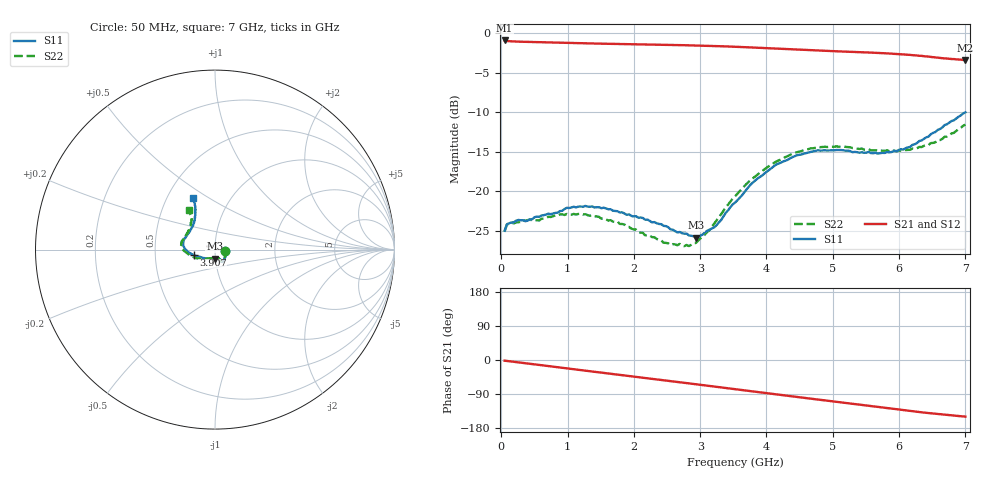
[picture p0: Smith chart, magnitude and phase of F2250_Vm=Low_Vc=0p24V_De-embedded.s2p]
! Integrated Device Technology
! Corporate Headquarters
! 6024 Silver Creek Valley Road
! San Jose, CA 95138  USA
! Phone:  1-408-284-8200
! Toll Free:  1-800-223-1366
! Webpage:  http://www.idt.com/
! Timing and RF Division
! 515 Groton Road, Suite 102
! Westford, MA 01886-6024
! Device:  F2250
! Description: Voltage Variable RF Attenuator
! Frequency:  50.0 -  6000.00 MHz
! Package:  3x3 mm Thin QFN Plastic Package: 16 pin
! Ports:  2 RF, 3 DC
!  Pin  1  = GND
!  Pin  2  = NC
!  Pin  3  = RF1  = Port 1
!  Pin  4  = NC
!  Pin  5  = GND
!  Pin  6  = GND
!  Pin  7  = GND
!  Pin  8  = GND
!  Pin  9  = NC
!  Pin 10  = RF2  = Port 2
!  Pin 11  = NC
!  Pin 12  = GND
!  Pin 13  = GND
!  Pin 14  = VCNTRL
!  Pin 15  = VDD
!  Pin 16  = VMODE
! Vcntrl:  0.240 Volts
! Vmode:  +0.000 Volts
! Vdd:  +3.30  Volts
! Current:  1.109 mA
! Data:  The device was measured on a the F2250 evaluation board which has
!  individual transmission lines to the RF pins.  Data was collected
!  using a calibrated network analyzer.  The evaluation board was
!  de-embedded using a TRL calibration technique.
!  The reference plane is the edge of the package pin.
! Misc:  SN 10
!  Action Tracker AT0258
! Date Measured:  2014-11-26
! Date:  2015-10-15  MJV
! Note:
!  Integrated Device Technology supplies this data as a sample of measured
!  data at the package pin for this product.  Your particular data for this
!  product may vary.
!  Data was taken at 25 degrees C.
!  Integrated Device Technology reserves the right to change this data at anytime.
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# GHz S dB R 50
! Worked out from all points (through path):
!   201 points, 50 MHz to 7 GHz, reference 50 ohm
!   highest |S21| = -0.93 dB at 50 MHz (marker M1); lowest = -3.4 dB at 7 GHz (marker M2)
!   group delay of S21, straight-line fit = 60 ps
!   lowest |S11| = -25.9 dB at 2.934 GHz (marker M3), VSWR 1.11, Z = 49.6 - j5.04 ohm
!   |S11| at or under -10 dB: start of sweep to end of sweep
!   |S22| runs from -27.0 to -11.6 dB; largest |S21 - S12| = 0.00036
!   S11 on the Smith chart (normalised r, x): 50 MHz: 1.12, -0.02; 3.907 GHz: 0.79, -0.05; 7 GHz: 0.67, +0.43
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0.05  -25.02 -9.6  -0.93 -1.8  -0.93 -1.8  -25.14 -10.1
0.08475  -24.20 -9.5  -1.00 -2.5  -1.00 -2.5  -24.26 -9.3
0.15425  -23.97 -11.8  -1.05 -4.0  -1.04 -4.0  -24.02 -11.0
0.57125  -23.26 -29.9  -1.15 -13.1  -1.15 -13.1  -23.74 -30.3
0.884  -22.55 -45.6  -1.21 -19.9  -1.21 -19.9  -22.98 -46.7
1.2315  -21.99 -55.8  -1.29 -27.4  -1.29 -27.4  -22.98 -59.6
1.75275  -22.56 -62.5  -1.38 -38.4  -1.38 -38.4  -23.86 -66.6
2.37825  -24.17 -63.3  -1.47 -51.8  -1.47 -51.8  -26.19 -67.9
2.552  -24.85 -67.5  -1.50 -55.6  -1.49 -55.6  -26.84 -73.4
2.83  -25.63 -82.8  -1.55 -61.7  -1.55 -61.7  -26.97 -92.7
2.93425  -25.89 -91.9  -1.57 -64.0  -1.57 -64.0  -26.58 -101.5
3.21225  -24.59 -121.5  -1.63 -70.1  -1.63 -70.1  -24.10 -127.5
3.525  -21.48 -147.9  -1.73 -77.1  -1.73 -77.1  -20.68 -146.3
3.76825  -19.11 -161.0  -1.82 -82.5  -1.82 -82.5  -18.54 -156.7
3.90725  -18.19 -165.4  -1.87 -85.5  -1.87 -85.5  -17.64 -162.8
4.1505  -16.63 -173.5  -1.97 -90.8  -1.97 -90.8  -16.25 -171.4
4.7065  -14.98 172.3  -2.18 -102.8  -2.18 -102.8  -14.58 175.6
5.15825  -14.84 161.6  -2.34 -112.6  -2.34 -112.6  -14.35 166.5
5.85325  -15.10 138.5  -2.59 -127.5  -2.59 -127.5  -14.96 151.5
6.166  -14.41 127.6  -2.76 -134.3  -2.76 -134.3  -14.78 142.6
6.444  -13.11 119.4  -2.97 -140.1  -2.97 -140.1  -14.16 133.3
7  -10.03 113.1  -3.41 -149.4  -3.41 -149.4  -11.59 123.8
